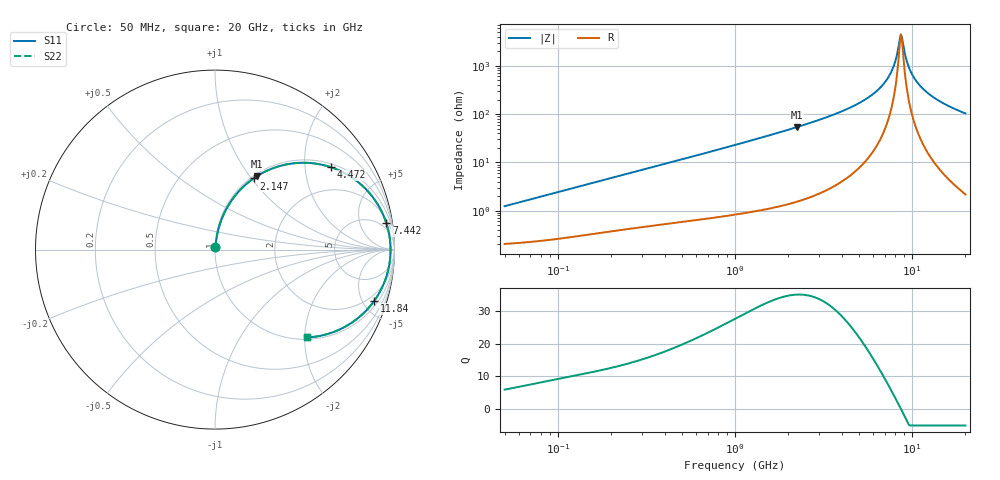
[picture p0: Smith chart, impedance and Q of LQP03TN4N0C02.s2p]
!Murata Part Number: LQP03TN4N0C02
!These Parameters are Measured in Series Mode Connection
!  o--[Z]--o
!Port1  Port2
!  o-------o
!Freq. Start=50[MHz] Stop=20[GHz], 401[Steps]
# Hz S RI R 50
!Freq.(Hz) S11(Real) S11(Imag) S21(Real) S21(Imag) S12(Real) S12(Imag) S22(Real) S22(Imag)
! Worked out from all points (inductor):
!   401 points, 50 MHz to 20 GHz, reference 50 ohm
!   read as one part in series: L = 3.87 nH near 51.52 MHz
!   highest Q = 35.1 at 2.245 GHz (marker M1), where L = 3.82 nH
!   self-resonance near 8.645 GHz
!   S11 on the Smith chart (normalised r, x): 50 MHz: 1.00, +0.02; 2.147 GHz: 1.03, +1.02; 4.472 GHz: 1.11, +2.72; 7.442 GHz: 3, +12; 11.84 GHz: 1.39, -6.07; 20 GHz: 1.04, -2.06
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5e7  0.00219 0.0121  0.9978 -0.0121  0.9978 -0.0121  0.00219 0.0121
1.364002e8  0.00408 0.0323  0.9959 -0.0323  0.9959 -0.0323  0.00408 0.0323
3.721004e8  0.0122 0.0844  0.9878 -0.0844  0.9878 -0.0844  0.0122 0.0844
1e9  0.0567 0.214  0.9433 -0.214  0.9433 -0.214  0.0567 0.214
2.146657e9  0.2145 0.3964  0.7855 -0.3964  0.7855 -0.3964  0.2145 0.3964
2.245319e9  0.2315 0.4078  0.7685 -0.4078  0.7685 -0.4078  0.2315 0.4078
2.728004e9  0.3194 0.452  0.6806 -0.452  0.6806 -0.452  0.3194 0.452
3.572216e9  0.4812 0.4838  0.5188 -0.4838  0.5188 -0.4838  0.4812 0.4838
4.472136e9  0.6442 0.4596  0.3558 -0.4596  0.3558 -0.4596  0.6442 0.4596
6.125241e9  0.8658 0.3088  0.1342 -0.3088  0.1342 -0.3088  0.8658 0.3088
6.802353e9  0.9208 0.2269  0.0792 -0.2269  0.0792 -0.2269  0.9208 0.2269
7.442007e9  0.9547 0.147  0.0453 -0.147  0.0453 -0.147  0.9547 0.147
7.901521e9  0.9693 0.0902  0.0307 -0.0902  0.0307 -0.0902  0.9693 0.0902
8.389408e9  0.977 0.0316  0.023 -0.0316  0.023 -0.0316  0.977 0.0316
8.644534e9  0.9781 0.00205  0.0219 -0.00205  0.0219 -0.00205  0.9781 0.00205
8.907419e9  0.9775 -0.0276  0.0225 0.0276  0.0225 0.0276  0.9775 -0.0276
9.316812e9  0.9731 -0.0717  0.0269 0.0717  0.0269 0.0717  0.9731 -0.0717
9.892087e9  0.9612 -0.1295  0.0388 0.1295  0.0388 0.1295  0.9612 -0.1295
1.066139e10  0.9369 -0.1983  0.0631 0.1983  0.0631 0.1983  0.9369 -0.1983
1.183995e10  0.8874 -0.2853  0.1126 0.2853  0.1126 0.2853  0.8874 -0.2853
1.482269e10  0.739 -0.4217  0.261 0.4217  0.261 0.4217  0.739 -0.4217
2e10  0.5149 -0.4893  0.4851 0.4893  0.4851 0.4893  0.5149 -0.4893
